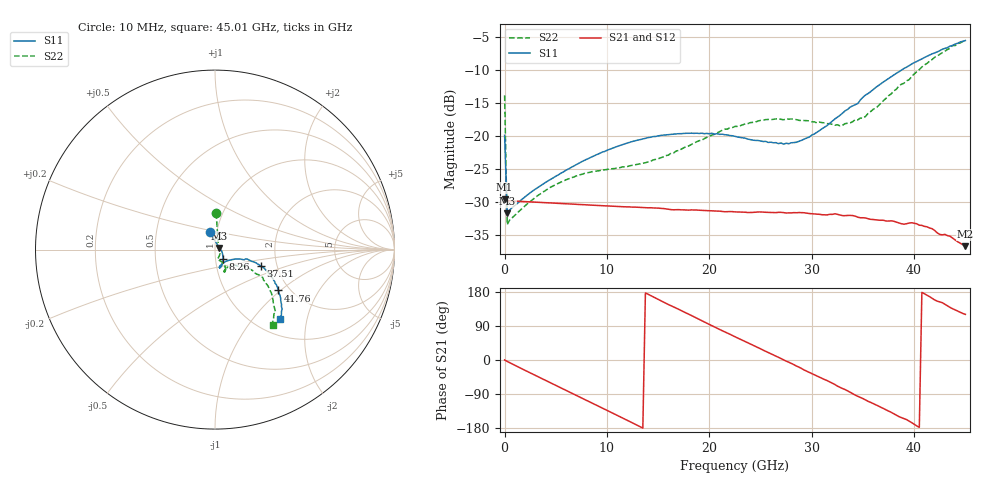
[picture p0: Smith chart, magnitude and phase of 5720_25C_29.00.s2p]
! Device:  ADRF5720
! Description: 0.5dB LSB GaAs MMIC 6-bit Digital Attenuator
! Frequency:  0.000009 -  40 GHz
! Ports:
!	RF1	= Port 1
!	RF2	= Port 2
! Vdd:  3.3 Volt
! Vss:  -3.3 Volt
! Control:  0/3.3 Volt
! State:  29.00 dB attenuation
! Data:  The device was measured using G-S-G Probes on a matrix board.
!  Data was collected using an calibrated 4 port network analyzer.
!  The reference plane for this measurement is at the launchers.
! Note:  Analog Devices supplies this data as a sample of measured data
!  for this product.  Your particular data for this product may vary.
!  Data was taken at 25 degrees C.
!  Analog Devices reserves the right to change this data at anytime.
# GHZ S DB R 45.0
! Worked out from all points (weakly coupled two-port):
!   181 points, 10 MHz to 45.01 GHz, reference 45 ohm
!   highest |S21| = -29.61 dB at 10 MHz (marker M1); lowest = -36.7 dB at 45.01 GHz (marker M2)
!   lowest |S11| = -31.7 dB at 260 MHz (marker M3), VSWR 1.05, Z = 47.2 + j0.883 ohm
!   |S11| at or under -10 dB: start of sweep to 38.76 GHz
!   |S22| runs from -33.4 to -5.5 dB; largest |S21 - S12| = 0.00018
!   S11 on the Smith chart (normalised r, x): 10 MHz: 0.93, +0.18; 8.26 GHz: 1.09, -0.11; 37.51 GHz: 1.65, -0.33; 41.76 GHz: 1.75, -0.97; 45.01 GHz: 1.30, -1.40
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0.01  -19.88 106.9  -29.61 0.1  -29.61 0.2  -13.84 88.2
0.26  -31.72 21.1  -29.81 -3.7  -29.81 -3.7  -33.44 22.5
1.26  -30.22 2.3  -29.88 -17.3  -29.88 -17.3  -31.62 -8.2
4.01  -27.03 -23.8  -30.09 -53.9  -30.09 -53.9  -28.23 -47.2
7.76  -23.72 -46.2  -30.41 -103.2  -30.41 -103.2  -25.69 -71.0
8.26  -23.36 -48.5  -30.46 -109.8  -30.46 -109.8  -25.52 -72.2
12.01  -21.05 -62.0  -30.74 -159.4  -30.74 -159.4  -24.62 -73.7
15.26  -19.90 -70.0  -30.97 156.5  -30.97 156.6  -23.29 -65.8
20.26  -19.58 -76.0  -31.35 90.4  -31.35 90.5  -19.86 -58.8
22.76  -20.14 -75.0  -31.51 58.2  -31.51 58.2  -18.53 -60.7
25.51  -20.81 -65.6  -31.56 22.8  -31.56 22.8  -17.50 -65.0
27.26  -21.23 -56.4  -31.61 -0.0  -31.61 0.0  -17.53 -66.3
30.26  -19.68 -33.5  -31.80 -38.9  -31.80 -38.9  -17.84 -65.7
32.76  -16.86 -21.4  -31.97 -72.1  -31.98 -72.1  -18.45 -56.1
33.76  -15.60 -19.6  -32.03 -85.1  -32.03 -85.1  -18.00 -47.8
35.01  -14.11 -17.0  -32.39 -101.8  -32.38 -101.8  -17.30 -40.3
37.51  -11.29 -19.8  -32.89 -134.6  -32.90 -134.5  -13.87 -29.3
37.76  -10.99 -20.4  -32.85 -138.0  -32.83 -137.9  -13.61 -28.8
40.26  -8.69 -27.4  -33.30 -173.9  -33.29 -173.9  -10.24 -30.3
41.76  -7.53 -32.8  -34.05 162.7  -34.05 162.8  -8.39 -36.5
43.76  -6.25 -40.5  -35.48 135.3  -35.51 135.1  -6.26 -46.0
45.01  -5.51 -46.5  -36.70 120.4  -36.73 120.4  -5.50 -52.6
